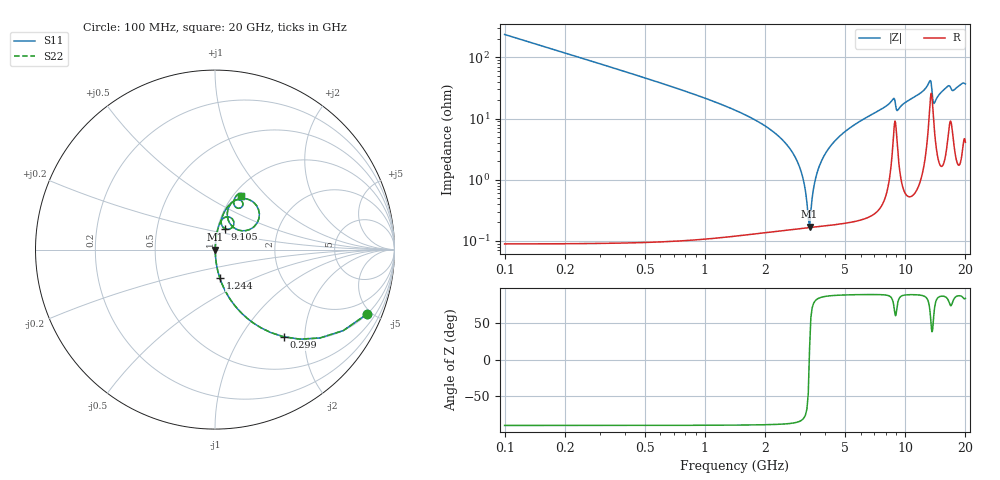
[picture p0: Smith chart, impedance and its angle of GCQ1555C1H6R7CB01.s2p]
!Murata Part Number: GCQ1555C1H6R7CB01
!These Parameters are Measured in Series Mode Connection
!Data Generated on Jan 08, 2026
!  o--ll--o
!Port1  Port2
!  o------o
!Operation Temp=25[degC], DC Bias Voltage=0[V]
!Freq. Start=100[MHz] Stop=20[GHz] 401[Steps]
# Hz S RI R 50
!Freq.(Hz) S11(Real) S11(Imag) S21(Real) S21(Imag) S12(Real) S12(Imag) S22(Real) S22(Imag)
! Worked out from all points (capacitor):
!   401 points, 100 MHz to 20 GHz, reference 50 ohm
!   read as one part in series: C = 6.7 pF near 199.5 MHz
!   lowest |Z| = 171 mohm at 3.334 GHz (marker M1)
!   series resonance near 3.323 GHz, so ESL is about 340 pH
!   S11 on the Smith chart (normalised r, x): 100 MHz: 1.00, -4.75; 299 MHz: 1.00, -1.58; 1.244 GHz: 1.00, -0.33; 9.105 GHz: 1.09, +0.26; 20 GHz: 1.08, +0.73
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1e8  0.8491 -0.3577  0.1509 0.3577  0.1509 0.3577  0.8491 -0.3577
2.99e8  0.3832 -0.4856  0.6168 0.4856  0.6168 0.4856  0.3832 -0.4856
5.975e8  0.1295 -0.3345  0.8705 0.3345  0.8705 0.3345  0.1295 -0.3345
1.24425e9  0.0273 -0.1594  0.9727 0.1594  0.9727 0.1594  0.0273 -0.1594
2.73675e9  0.00231 -0.0279  0.9977 0.0279  0.9977 0.0279  0.00231 -0.0279
3.03525e9  0.00176 -0.013  0.9982 0.013  0.9982 0.013  0.00176 -0.013
3.23425e9  0.00164 -0.00389  0.9984 0.00389  0.9984 0.00389  0.00164 -0.00389
3.33375e9  0.00165 0.000445  0.9984 -0.000445  0.9984 -0.000445  0.00165 0.000445
3.43325e9  0.00169 0.00465  0.9983 -0.00465  0.9983 -0.00465  0.00169 0.00465
3.53275e9  0.00176 0.00874  0.9982 -0.00874  0.9982 -0.00874  0.00176 0.00874
3.73175e9  0.00199 0.0166  0.998 -0.0166  0.998 -0.0166  0.00199 0.0166
4.279e9  0.00315 0.0366  0.9968 -0.0366  0.9968 -0.0366  0.00315 0.0366
6.7665e9  0.0155 0.1131  0.9845 -0.1131  0.9845 -0.1131  0.0155 0.1131
8.70675e9  0.0753 0.1821  0.9247 -0.1821  0.9247 -0.1821  0.0753 0.1821
9.10475e9  0.0567 0.1157  0.9433 -0.1157  0.9433 -0.1157  0.0567 0.1157
1.005e10  0.0382 0.1765  0.9618 -0.1765  0.9618 -0.1765  0.0382 0.1765
1.248775e10  0.0953 0.2635  0.9047 -0.2635  0.9047 -0.2635  0.0953 0.2635
1.338325e10  0.2424 0.2236  0.7576 -0.2236  0.7576 -0.2236  0.2424 0.2236
1.39305e10  0.0941 0.1315  0.9059 -0.1315  0.9059 -0.1315  0.0941 0.1315
1.507475e10  0.0788 0.2397  0.9212 -0.2397  0.9212 -0.2397  0.0788 0.2397
1.67165e10  0.1553 0.2556  0.8447 -0.2556  0.8447 -0.2556  0.1553 0.2556
2e10  0.1454 0.3011  0.8546 -0.3011  0.8546 -0.3011  0.1454 0.3011
